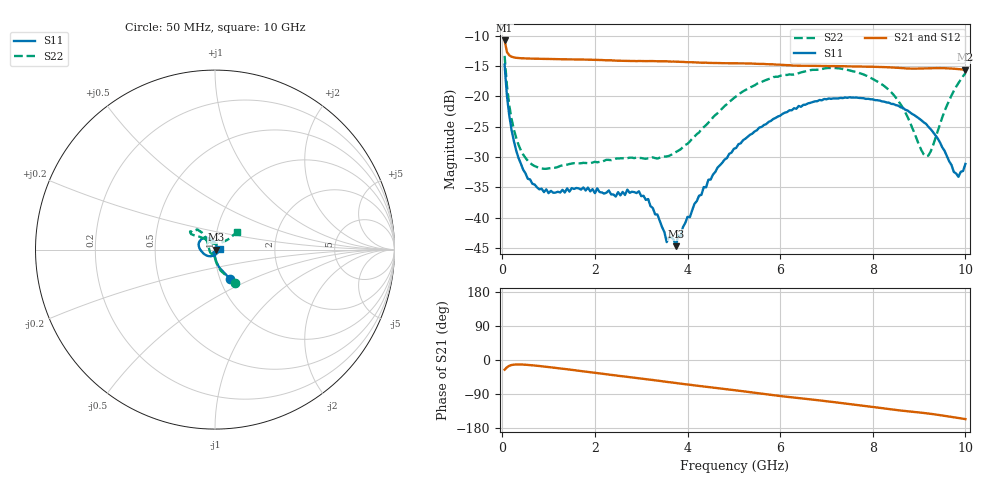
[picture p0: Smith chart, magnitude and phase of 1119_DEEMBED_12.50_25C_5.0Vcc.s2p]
!Hittite Microwave Corp.
!Digital Attenuator/PhaseShifter Rev 1.4.0
!Filename: C:\DATA\DATA\1119_DEEMBED_12.50_25C_5.0Vcc.s2p
!VNA ID: Agilent Technologies,N5224A,MY51441122,A.10.45.03
!Device type:
!2 Port Calibration.
!Temp(C): 25
!Lot Number:
!Serial Number:
!Operator:
!Misc:
!Attenuator:  12.500
# GHZ S DB R 50.0
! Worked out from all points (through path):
!   200 points, 50 MHz to 10 GHz, reference 50 ohm
!   highest |S21| = -10.78 dB at 50 MHz (marker M1); lowest = -15.6 dB at 10 GHz (marker M2)
!   group delay of S21, straight-line fit = 41.2 ps
!   lowest |S11| = -44.7 dB at 3.75 GHz (marker M3), VSWR 1.01, Z = 50.6 + j0.000308 ohm
!   |S11| at or under -10 dB: start of sweep to end of sweep
!   |S22| runs from -31.9 to -13.3 dB; largest |S21 - S12| = 0.00053
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0.05  -14.76 -62.9  -10.78 -25.5  -10.78 -25.5  -13.32 -59.6
0.1  -19.90 -77.0  -12.68 -19.3  -12.67 -19.2  -18.23 -74.7
0.2  -25.55 -86.9  -13.46 -13.3  -13.46 -13.3  -23.73 -85.8
0.35  -30.16 -93.2  -13.68 -11.7  -13.68 -11.7  -27.98 -92.5
0.55  -33.59 -100.4  -13.76 -12.9  -13.76 -12.9  -30.62 -98.3
1  -35.96 -109.6  -13.83 -18.6  -13.83 -18.6  -31.87 -106.2
1.75  -35.02 -115.1  -13.93 -29.9  -13.93 -29.9  -30.97 -114.6
2.45  -36.53 -102.8  -14.11 -40.8  -14.11 -40.9  -30.26 -133.3
2.95  -35.66 -90.1  -14.17 -48.0  -14.18 -48.1  -30.15 -151.8
3.4  -40.54 -72.7  -14.21 -55.1  -14.21 -55.2  -30.12 -174.1
3.55  -44.04 -43.1  -14.22 -57.7  -14.23 -57.8  -29.91 177.3
3.65  -43.25 -26.0  -14.27 -59.1  -14.28 -59.1  -29.63 172.2
3.75  -44.71 0.0  -14.28 -60.8  -14.29 -60.8  -29.20 166.5
4.35  -34.96 56.4  -14.44 -69.8  -14.46 -69.8  -25.07 137.6
5.05  -28.51 89.9  -14.55 -80.2  -14.57 -80.2  -20.00 126.8
6.7  -20.95 134.2  -14.96 -104.6  -14.97 -104.6  -15.63 139.9
7.65  -20.20 157.4  -15.07 -118.5  -15.08 -118.6  -15.99 146.9
8.35  -21.04 172.8  -15.21 -129.4  -15.21 -129.4  -18.96 140.4
8.65  -21.88 -177.3  -15.35 -134.1  -15.35 -134.1  -21.91 133.3
9.15  -24.53 -147.6  -15.38 -140.4  -15.39 -140.5  -29.90 90.2
9.85  -33.27 -34.1  -15.49 -153.1  -15.50 -153.1  -17.80 38.2
10  -31.15 6.0  -15.60 -155.9  -15.61 -155.9  -16.19 39.3
